| TEXAS INSTRUMENTS INCORPORATED
| Standard Linear and Logic Group
| IBIS Model of TS5A2053
| SINGLE CHANNEL 10-OHM SPDT ANALOG SWITCH WITH ENABLE
| This file contains package information for the following:
|  SOT 8-pin (DCT) package as [Component] TS5A2053_DCT
|  DSBGA 8-pin (YEP_YZP) package as [Component] TS5A2053_YEP_YZP
|  SOT 8-pin (DCU) package as [Component] TS5A2053_DCU
| This device can be Powered at the following Vccs:
|  1.8 volt Vcc
|  2.5 volt Vcc
|  3.3 volt Vcc
|  5 volt Vcc
| This file provides unique models under the [Model Selector] for each Vcc.
| For operation at a specific Vcc, select the appropriate model after each
| [Model Selector] keyword.
[IBIS Ver]   3.2
[Comment char]  |_char
[File Name]   ts5a2053.ibs
[File Rev]   1.1 | x_die
[Date]   January 6, 2005
[Source]   Data created from TI-SPICE simulations at TI-SLL.
[Notes]   The following is an IBIS list for the TS5A2053.
   Please contact sllibis@ti.com with questions and
   comments concerning SLL IBIS models.
   - FILE REV HISTORY
   - 1.1 Release IBIS file on 01/25/05
   - Power clamp data deleted in the IN and NEN models as there
   is no power-clamp diode.
   - Non-monotonic data due to FET characteristics.
   - NCH & PCH MOSFETS, so [Series Mosfet] model can have rising
   or falling currents
   - YEP and YZP packages are package preview only at this date.
[Disclaimer] Property of Texas Instruments Incorporated.  Unauthorized
   reproduction and/or distribution is strictly prohibited.
   This product is protected under copyright law.
   Created  2005, (C) Copyright  2005, Texas Instruments
   Incorporated, All Rights Reserved
   UNLESS THERE IS A SIGNED, WRITTEN AGREEMENT TO THE
   CONTRARY, TEXAS INSTRUMENTS (TI) IS PROVIDING THE IBIS
   MODELS  AND WITHOUT ANY WARRANTY, EXPRESSED OR
   IMPLIED.  TI assumes no liability for:
   1) the accuracy of the IBIS models provided to your
   company;
   2) the proper functioning of these IBIS Models in your
   design or for any resulting applications; or
   3) infringement of patents, copyrights or intellectual
   property rights resulting from your use of these IBIS
   models.
   TI provides IBIS Models as a service to our customers.
   You and your company shall not distribute, sell or give
   these models to anyone else without prior written
   permission from TI.
   TI reserves the right to make changes to our products or
   to discontinue any semiconductor product or service
   without notice, and advises our customers to obtain the
   latest version of relevant information to verify, before
   placing orders, that the information being relied on is
   current.
   Please be aware that your receipt and use of the IBIS
   information provided shall serve as acceptance of these
   terms and conditions.  If you do not accept these terms,
   you should return or destroy the IBIS models and any
   other accompanying information immediately.
| Component TS5A2053_DCT 8-pin SOT
[Component]   TS5A2053_DCT
[Manufacturer]   Texas Instruments, Inc.
[Package]
|   typ   min   max
R_pkg   2.900e-02   2.800e-02   3.100e-02
L_pkg   1.796e-09   1.666e-09   1.924e-09
C_pkg   2.310e-13   2.210e-13   2.420e-13
[Pin]   signal_name   model_name   R_pin   L_pin   C_pin
1   COM   TS5A2053_COM   3.100e-02   1.894e-09   2.230e-13
2   NEN   TS5A2053_NEN   2.800e-02   1.697e-09   2.370e-13
3   GND   GND   3.000e-02   1.722e-09   2.390e-13
4   GND   GND   3.000e-02   1.861e-09   2.210e-13
5   IN   TS5A2053_IN   2.800e-02   1.924e-09   2.280e-13
6   NO   TS5A2053_NONC   2.900e-02   1.736e-09   2.420e-13
7   NC   TS5A2053_NONC   2.800e-02   1.666e-09   2.360e-13
8   VPLUS   POWER   3.000e-02   1.871e-09   2.220e-13
| Component TS5A2053_YEP_YZP 8-pin DSBGA
[Component]   TS5A2053_YEP_YZP
[Manufacturer]   Texas Instruments, Inc.
[Package]
|   typ   min   max
R_pkg   1.000e-03   1.000e-03   4.000e-03
L_pkg   6.400e-11   2.400e-11   3.790e-10
C_pkg   5.800e-14   0.000e+00   6.700e-14
[Pin]   signal_name   model_name   R_pin   L_pin   C_pin
1   COM   TS5A2053_COM   1.000e-03   2.500e-11   6.400e-14
2   NEN   TS5A2053_NEN   1.000e-03   2.400e-11   6.700e-14
3   GND   GND   1.000e-03   2.400e-11   6.700e-14
4   GND   GND   1.000e-03   2.500e-11   6.400e-14
5   IN   TS5A2053_IN   1.000e-03   2.500e-11   6.400e-14
6   NO   TS5A2053_NONC   1.000e-03   2.400e-11   6.700e-14
7   NC   TS5A2053_NONC   1.000e-03   2.400e-11   6.700e-14
8   VPLUS   POWER   1.000e-03   2.500e-11   6.400e-14
| Component TS5A2053_DCU 8-pin SOT
[Component]   TS5A2053_DCU
[Manufacturer]   Texas Instruments, Inc.
[Package]
|   typ   min   max
R_pkg   2.600e-02   2.300e-02   3.800e-02
L_pkg   1.394e-09   1.066e-09   2.046e-09
C_pkg   2.590e-13   2.150e-13   3.720e-13
[Pin]   signal_name   model_name   R_pin   L_pin   C_pin
1   COM   TS5A2053_COM   2.400e-02   1.520e-09   2.710e-13
2   NEN   TS5A2053_NEN   2.300e-02   1.112e-09   2.180e-13
3   GND   GND   2.300e-02   1.070e-09   2.170e-13
4   GND   GND   2.700e-02   2.046e-09   3.720e-13
5   IN   TS5A2053_IN   2.700e-02   1.542e-09   2.730e-13
6   NO   TS5A2053_NONC   2.300e-02   1.100e-09   2.240e-13
7   NC   TS5A2053_NONC   2.300e-02   1.066e-09   2.150e-13
8   VPLUS   POWER   3.800e-02   1.696e-09   2.800e-13
[Series Switch Groups]
| Function Group States
On  1 /   | COM->NC NEN LOW, IN LOW
On  2 /   | COM->NO NEN LOW, IN HIGH
On  3 /   | NC->COM NEN LOW, IN LOW
On  4 /   | NO->COM NEN LOW, IN HIGH
Off 1 2 3 4 /   | NEN HIGH
[Series Pin Mapping]   pin_2   model_name   function_table_group
1   7   TS5A2053_COM_18_S   1
| 1   7   TS5A2053_COM_25_S   1
| 1   7   TS5A2053_COM_33_S   1
| 1   7   TS5A2053_COM_50_S   1
1   6   TS5A2053_COM_18_S   2
| 1   6   TS5A2053_COM_25_S   2
| 1   6   TS5A2053_COM_33_S   2
| 1   6   TS5A2053_COM_50_S   2
7   1   TS5A2053_NONC_18_S   3
| 7   1   TS5A2053_NONC_25_S   3
| 7   1   TS5A2053_NONC_33_S   3
| 7   1   TS5A2053_NONC_50_S   3
6   1   TS5A2053_NONC_18_S   4
| 6   1   TS5A2053_NONC_25_S   4
| 6   1   TS5A2053_NONC_33_S   4
| 6   1   TS5A2053_NONC_50_S   4
| Model TS5A2053_NEN
[Model Selector]   TS5A2053_NEN
TS5A2053_NEN_18   1.8 volt Vcc
TS5A2053_NEN_25   2.5 volt Vcc
TS5A2053_NEN_33   3.3 volt Vcc
TS5A2053_NEN_50   5 volt Vcc
| Model TS5A2053_IN
[Model Selector]   TS5A2053_IN
TS5A2053_IN_18   1.8 volt Vcc
TS5A2053_IN_25   2.5 volt Vcc
TS5A2053_IN_33   3.3 volt Vcc
TS5A2053_IN_50   5 volt Vcc
| Model TS5A2053_COM
[Model Selector]   TS5A2053_COM
TS5A2053_COM_18   1.8 volt Vcc
TS5A2053_COM_25   2.5 volt Vcc
TS5A2053_COM_33   3.3 volt Vcc
TS5A2053_COM_50   5 volt Vcc
| Model TS5A2053_COM_S
[Model Selector]   TS5A2053_COM_S
TS5A2053_COM_18_S   1.8 volt Vcc_S
TS5A2053_COM_25_S   2.5 volt Vcc_S
TS5A2053_COM_33_S   3.3 volt Vcc_S
TS5A2053_COM_50_S   5 volt Vcc_S
| Model TS5A2053_NONC
[Model Selector]   TS5A2053_NONC
TS5A2053_NONC_18   1.8 volt Vcc
TS5A2053_NONC_25   2.5 volt Vcc
TS5A2053_NONC_33   3.3 volt Vcc
TS5A2053_NONC_50   5 volt Vcc
| Model TS5A2053_NONC_S
[Model Selector]   TS5A2053_NONC_S
TS5A2053_NONC_18_S   1.8 volt Vcc_S
TS5A2053_NONC_25_S   2.5 volt Vcc_S
TS5A2053_NONC_33_S   3.3 volt Vcc_S
TS5A2053_NONC_50_S   5 volt Vcc_S
[Model]   TS5A2053_COM_18_S
Model_type  Series_switch
| variable   typ   min   max
C_comp   0   0   0
[Temperature Range]   40   100   -40
| Ambient temperature   25   85   -40
[Voltage range]   1.8   1.65   1.95
[On]
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[Off]
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[Model]   TS5A2053_COM_25_S
Model_type  Series_switch
| variable   typ   min   max
C_comp   0   0   0
[Temperature Range]   40   100   -40
| Ambient temperature   25   85   -40
[Voltage range]   2.5   2.3   2.7
[On]
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[Off]
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[Model]   TS5A2053_COM_33_S
Model_type  Series_switch
| variable   typ   min   max
C_comp   0   0   0
[Temperature Range]   40   100   -40
| Ambient temperature   25   85   -40
[Voltage range]   3.3   3   3.6
[On]
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[Off]
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[Model]   TS5A2053_COM_50_S
Model_type  Series_switch
| variable   typ   min   max
C_comp   0   0   0
[Temperature Range]   40   100   -40
| Ambient temperature   25   85   -40
[Voltage range]   5   4.5   5.5
[On]
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[Off]
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[Model]   TS5A2053_NONC_18_S
Model_type  Series_switch
| variable   typ   min   max
C_comp   0   0   0
[Temperature Range]   40   100   -40
| Ambient temperature   25   85   -40
[Voltage range]   1.8   1.65   1.95
[On]
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[Off]
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[Model]   TS5A2053_NONC_25_S
Model_type  Series_switch
| variable   typ   min   max
C_comp   0   0   0
[Temperature Range]   40   100   -40
| Ambient temperature   25   85   -40
[Voltage range]   2.5   2.3   2.7
[On]
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[Off]
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[Model]   TS5A2053_NONC_33_S
Model_type  Series_switch
| variable   typ   min   max
C_comp   0   0   0
[Temperature Range]   40   100   -40
| Ambient temperature   25   85   -40
[Voltage range]   3.3   3   3.6
[On]
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[Off]
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[Model]   TS5A2053_NONC_50_S
Model_type  Series_switch
| variable   typ   min   max
C_comp   0   0   0
[Temperature Range]   40   100   -40
| Ambient temperature   25   85   -40
[Voltage range]   5   4.5   5.5
[On]
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[Off]
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| Models and submodels in the file (24): TS5A2053_NEN_18 (Input), TS5A2053_NEN_25 (Input), TS5A2053_NEN_33 (Input), TS5A2053_NEN_50 (Input), TS5A2053_IN_18 (Input), TS5A2053_IN_25 (Input), TS5A2053_IN_33 (Input), TS5A2053_IN_50 (Input), TS5A2053_COM_18_S (Series_switch), TS5A2053_COM_18 (Terminator), TS5A2053_COM_25_S (Series_switch), TS5A2053_COM_25 (Terminator), TS5A2053_COM_33_S (Series_switch), TS5A2053_COM_33 (Terminator), TS5A2053_COM_50_S (Series_switch), TS5A2053_COM_50 (Terminator), TS5A2053_NONC_18_S (Series_switch), TS5A2053_NONC_18 (Terminator), TS5A2053_NONC_25_S (Series_switch), TS5A2053_NONC_25 (Terminator), TS5A2053_NONC_33_S (Series_switch), TS5A2053_NONC_33 (Terminator), TS5A2053_NONC_50_S (Series_switch), TS5A2053_NONC_50 (Terminator)
